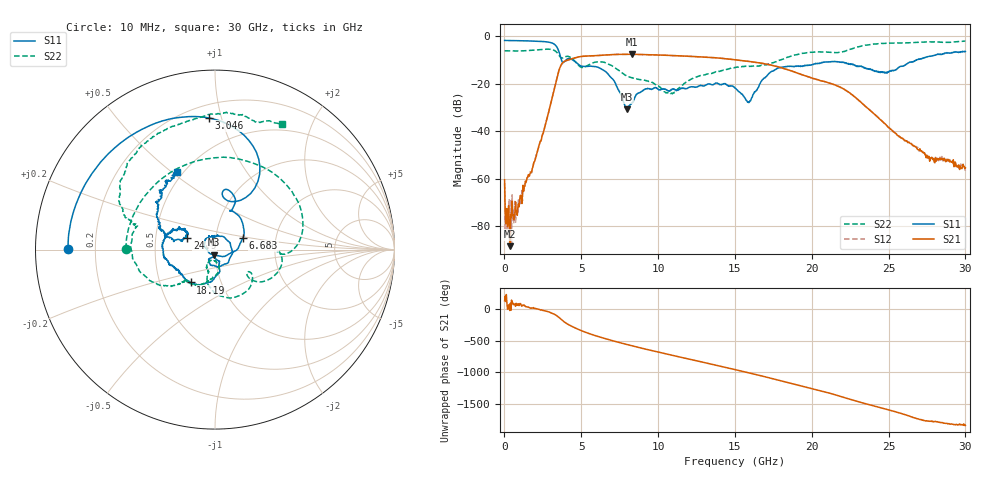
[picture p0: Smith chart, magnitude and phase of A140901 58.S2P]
!  2-Port S-parameters saved by WinCal
! VAR MeasName=S-Parameters (CALIBRATED_DATA) read from VNA (N5244A)
! VAR MeasDate=11/3/2014 9:36:28 AM
! VAR NAME=A140901 58
! VAR FILENAME=A140901 58.S2P
! VAR DATE=11/3/2014 9:36:28 AM
! VAR PHYS_PORTS=1,2
# Hz S RI R 50
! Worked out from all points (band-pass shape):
!   801 points, 10 MHz to 30 GHz, reference 50 ohm
!   highest |S21| = -7.56 dB at 8.295 GHz (marker M1); lowest = -88.5 dB at 347.4 MHz (marker M2)
!   |S21| within 3 dB of the highest: 3.893 GHz to 15.9 GHz (12.01 GHz wide, 121 % of centre)
!   lowest |S11| = -30.7 dB at 7.957 GHz (marker M3), VSWR 1.06, Z = 49.3 - j2.82 ohm
!   |S11| at or under -10 dB: 3.713 GHz to 4 GHz (287.1 MHz wide, 7.44 % of centre); 4.457 GHz to 26.78 GHz (22.32 GHz wide, 143 % of centre); 26.77756 GHz to 26.82444 GHz (46.88 MHz wide, 0.175 % of centre)
!   |S22| runs from -24.2 to -2.0 dB; largest |S21 - S12| = 0.0024
!   S11 on the Smith chart (normalised r, x): 10 MHz: 0.10, +0.00; 3.046 GHz: 0.29, +0.91; 6.683 GHz: 1.35, +0.18; 18.19 GHz: 0.72, -0.28; 24.9 GHz: 0.73, +0.10; 30 GHz: 0.47, +0.52
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1e7  -0.8197 0.00315  -0.000684 0.000652  0.000117 -0.000784  -0.4961 0.00394
3.473875e8  -0.8107 0.1132  3.56e-05 -1.22e-05  0.000135 0.000219  -0.4717 0.1481
8.722125e8  -0.7637 0.2788  9.95e-05 0.00023  0.000107 0.000161  -0.3621 0.3323
2.071812e9  -0.5034 0.6115  0.00295 0.000506  0.00316 0.000583  0.0852 0.5128
3.046488e9  -0.0322 0.733  0.0242 -0.035  0.0242 -0.0351  0.4711 0.2465
3.75875e9  0.1163 0.268  -0.2693 -0.0288  -0.2689 -0.0288  0.3473 -0.011
4.35855e9  0.0929 0.317  -0.0161 0.3345  -0.0157 0.3338  0.3107 -0.1607
5.033325e9  0.089 0.2173  0.3591 0.1181  0.3588 0.118  0.1779 -0.1316
6.682775e9  0.1555 0.0647  -0.1667 -0.3703  -0.166 -0.37  0.0485 -0.2629
7.95735e9  -0.00592 -0.0286  -0.3959 0.1352  -0.3959 0.134  -0.0427 -0.1397
8.294738e9  -0.0375 -0.0121  -0.3217 0.2685  -0.3211 0.2679  -0.0373 -0.1292
1.001916e10  -0.0271 0.072  0.3144 0.2554  0.3134 0.2547  -0.0456 -0.0771
1.095635e10  -0.00408 0.0782  0.3828 -0.091  0.3831 -0.0904  0.000253 -0.0631
1.23059e10  0.0556 0.0651  0.0148 -0.3752  0.0147 -0.3755  0.0145 -0.1314
1.369294e10  0.0757 -0.0656  -0.3422 -0.0924  -0.3414 -0.0926  -0.0311 -0.1715
1.5005e10  -0.0299 -0.0754  -0.1665 0.2745  -0.1656 0.2742  -0.0979 -0.1975
1.59047e10  -0.00594 -0.0396  0.1028 0.2782  0.1021 0.2784  -0.1463 -0.1837
1.819144e10  -0.1355 -0.1829  0.0749 -0.1951  0.0755 -0.1954  -0.2697 -0.2015
2.002832e10  -0.2366 -0.09  -0.1317 0.00285  -0.1321 0.00177  -0.4606 -0.0283
2.49017e10  -0.1547 0.0641  -0.0114 -0.00601  -0.0113 -0.00616  -0.349 0.6246
2.501416e10  -0.1629 0.0644  -0.0111 -0.00429  -0.0111 -0.00453  -0.3327 0.6385
3e10  -0.2089 0.4323  0.00114 -0.00124  0.00112 -0.000933  0.3743 0.7014
